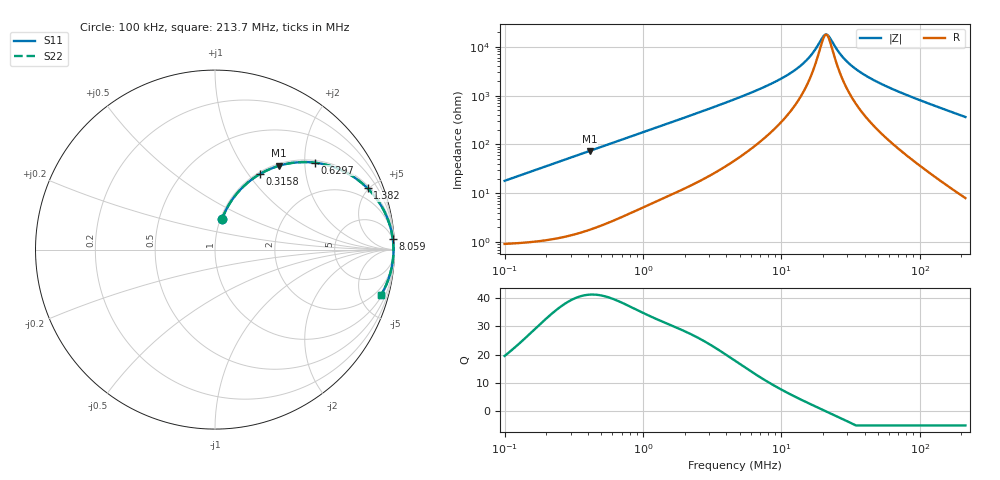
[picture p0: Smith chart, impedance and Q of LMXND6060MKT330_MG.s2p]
! LMXND6060MKT330_MG  S-PARAMETER MODEL  ( General Type )
! Model Generated by TAIYO YUDEN Corporation (http://www.ty-top.com)
! Version 1.0
! TAIYO YUDEN Control No. 191025NI43SB-FBB
! Copyright(c) 2019 TAIYO YUDEN CO.,LTD. All Rights Reserved.
! Product Description (link to TY-COMPAS)
! https://ds.yuden.co.jp/TYCOMPAS/or/detail?pn=LMXND6060MKT330MMG&u=M
! Products Name : Inductors
! Characteristics :
!  Inductance : 33 uH , SRF(min) : 8.0 MHz , DC Resistance(max) : 0.696 Ohm
!  Rated Current : Saturation :590 mA , Temp Rise : 550 mA
!  Case Size : 6.0 x 6.0 / 0.236 x 0.236 [mm/inch] , Thickness : 1.2 / 0.047 [mm/inch]
!  (Conditions: Temperature = 25 degC , DC Bias Current/Voltage = 0A / 0V)
! External Node Assignments :
!  1  o---GGG---o  2
! GND o---------o GND
! Frequency Range : 0.1MHz  -  213.673535MHz  [ 402 STEP ]
# MHz S RI R 50
! Freq[MHz].  S11 Real  S11 Imag  S21 Real  S21 Imag  S12 Real  S12 Imag  S22 Real  S22 Imag
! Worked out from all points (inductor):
!   401 points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, 100 kHz to 213.7 MHz, reference 50 ohm
!   read as one part in series: L = 28.6 uH near 103.9 kHz
!   highest Q = 41.2 at 413.1 kHz (marker M1), where L = 28.5 uH
!   self-resonance near 21.01 MHz
!   S11 on the Smith chart (normalised r, x): 100 kHz: 1.02, +0.36; 315.8 kHz: 1.03, +1.13; 629.7 kHz: 1.06, +2.25; 1.382 MHz: 1.15, +4.90; 8.059 MHz: 4, +33; 213.7 MHz: 1.16, -7.30
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0.1  0.0397 0.1713  0.9603 -0.1713  0.9603 -0.1713  0.0397 0.1713
0.188237  0.1101 0.2976  0.8899 -0.2976  0.8899 -0.2976  0.1101 0.2976
0.315837  0.2485 0.4197  0.7515 -0.4197  0.7515 -0.4197  0.2485 0.4197
0.361188  0.3 0.4462  0.7 -0.4462  0.7 -0.4462  0.3 0.4462
0.413051  0.3573 0.4672  0.6427 -0.4672  0.6427 -0.4672  0.3573 0.4672
0.629709  0.5575 0.4842  0.4425 -0.4842  0.4425 -0.4842  0.5575 0.4842
1.304567  0.8354 0.3556  0.1646 -0.3556  0.1646 -0.3556  0.8354 0.3556
1.381782  0.8498 0.3418  0.1502 -0.3418  0.1502 -0.3418  0.8498 0.3418
2.363318  0.939 0.2213  0.061 -0.2213  0.061 -0.2213  0.939 0.2213
4.71194  0.9806 0.1123  0.0194 -0.1123  0.0194 -0.1123  0.9806 0.1123
8.059021  0.9905 0.0597  0.00947 -0.0597  0.00947 -0.0597  0.9905 0.0597
12.524  0.9935 0.0292  0.00652 -0.0292  0.00652 -0.0292  0.9935 0.0292
14.5995  0.994 0.0201  0.00604 -0.0201  0.00604 -0.0201  0.994 0.0201
16.69585  0.9942 0.0126  0.00576 -0.0126  0.00576 -0.0126  0.9942 0.0126
19.83938  0.9944 0.00317  0.00559 -0.00317  0.00559 -0.00317  0.9944 0.00317
21.4203  0.9944 -0.000963  0.00557 0.000963  0.00557 0.000963  0.9944 -0.000963
22.25739  0.9944 -0.00303  0.00558 0.00303  0.00558 0.00303  0.9944 -0.00303
26.95988  0.9943 -0.0135  0.00574 0.0135  0.00574 0.0135  0.9943 -0.0135
32.03594  0.9939 -0.0233  0.0061 0.0233  0.0061 0.0233  0.9939 -0.0233
41.89659  0.9928 -0.04  0.00716 0.04  0.00716 0.04  0.9928 -0.04
60.30341  0.9898 -0.0675  0.0102 0.0675  0.0102 0.0675  0.9898 -0.0675
213.6735  0.9255 -0.2519  0.0745 0.2519  0.0745 0.2519  0.9255 -0.2519
